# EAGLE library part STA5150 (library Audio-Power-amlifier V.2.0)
200W MONO POWER AMPLIFIER. The STA5150 is a fully integrated power module designed to implement a BASH® amplifier when used in conjunction with STABP01 digital processor.
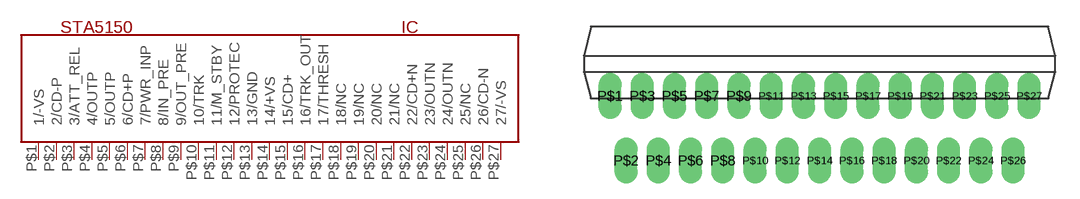
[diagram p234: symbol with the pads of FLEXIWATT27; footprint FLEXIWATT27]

Designator prefix IC

## STA5150  [FLEXIWATT27]
P$1  1/-VS  pwr
P$2  2/CD-P  pwr
P$3  3/ATT_REL
P$4  4/OUTP  out
P$5  5/OUTP  out
P$6  6/CD+P  pwr
P$7  7/PWR_INP  in
P$8  8/IN_PRE  in
P$9  9/OUT_PRE  out
P$10  10/TRK  in
P$11  11/M_STBY  in
P$12  12/PROTEC
P$13  13/GND  pwr
P$14  14/+VS  pwr
P$15  15/CD+  pwr
P$16  16/TRK_OUT  out
P$17  17/THRESH  in
P$18  18/NC  nc
P$19  19/NC  nc
P$20  20/NC  nc
P$21  21/NC  nc
P$22  22/CD+N  pwr
P$23  23/OUTN  out
P$24  24/OUTN  out
P$25  25/NC  nc
P$26  26/CD-N  pwr
P$27  27/-VS  pwr

## Footprint FLEXIWATT27 (pad centres in mm)
Flexiwatt27
drill 0.7 pad 1.422 long: P$1 -13,0; P$2 -12,-4; P$3 -11,0; P$4 -10,-4; P$5 -9,0; P$6 -8,-4; P$7 -7,0; P$8 -6,-4; P$9 -5,0; P$10 -4,-4; P$11 -3,0; P$12 -2,-4; P$13 -1,0; P$14 0,-4; P$15 1,0; P$16 2,-4; P$17 3,0; P$18 4,-4; P$19 5,0; P$20 6,-4; P$21 7,0; P$22 8,-4; P$23 9,0; P$24 10,-4; P$25 11,0; P$26 12,-4; P$27 13,0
